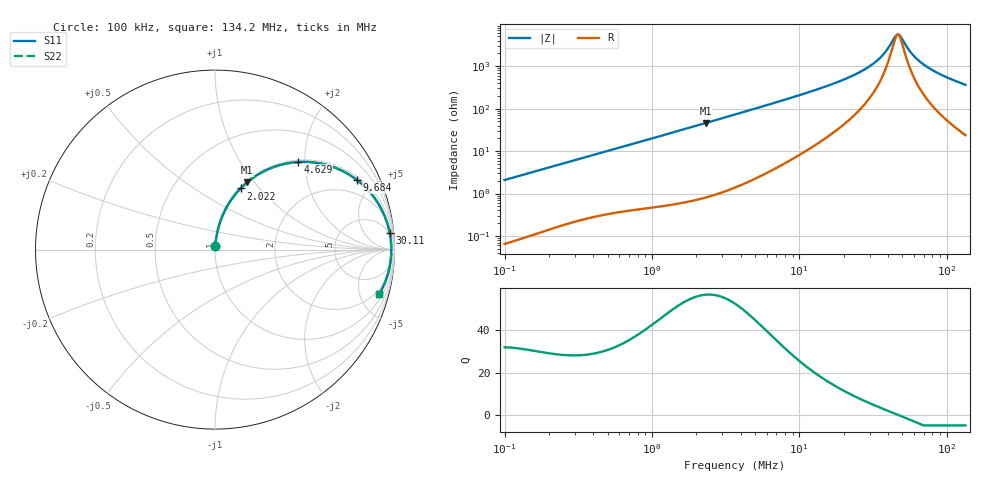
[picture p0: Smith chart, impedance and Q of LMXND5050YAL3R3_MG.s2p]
! LMXND5050YAL3R3_MG  S-PARAMETER MODEL  ( General Type )
! Model Generated by TAIYO YUDEN Corporation (http://www.ty-top.com)
! Version 1.0
! TAIYO YUDEN Control No. 191023NI43SB-FBB
! Copyright(c) 2019 TAIYO YUDEN CO.,LTD. All Rights Reserved.
! Product Description (link to TY-COMPAS)
! https://ds.yuden.co.jp/TYCOMPAS/or/detail?pn=LMXND5050YAL3R3NMG&u=M
! Products Name : Inductors
! Characteristics :
!  Inductance : 3.3 uH , SRF(min) : 32 MHz , DC Resistance(max) : 0.0351 Ohm
!  Rated Current : Saturation :4000 mA , Temp Rise : 3300 mA
!  Case Size : 4.9 x 4.9 / 0.193 x 0.193 [mm/inch] , Thickness : 4.1 / 0.161 [mm/inch]
!  (Conditions: Temperature = 25 degC , DC Bias Current/Voltage = 0A / 0V)
! External Node Assignments :
!  1  o---GGG---o  2
! GND o---------o GND
! Frequency Range : 0.1MHz  -  134.160692MHz  [ 402 STEP ]
# MHz S RI R 50
! Freq[MHz].  S11 Real  S11 Imag  S21 Real  S21 Imag  S12 Real  S12 Imag  S22 Real  S22 Imag
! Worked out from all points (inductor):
!   401 points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, 100 kHz to 134.2 MHz, reference 50 ohm
!   read as one part in series: L = 3.31 uH near 103.7 kHz
!   highest Q = 56.8 at 2.335 MHz (marker M1), where L = 3.15 uH
!   self-resonance near 46.38 MHz
!   S11 on the Smith chart (normalised r, x): 100 kHz: 1.00, +0.04; 2.022 MHz: 1.01, +0.80; 4.629 MHz: 1.04, +1.84; 9.684 MHz: 1.15, +3.98; 30.11 MHz: 5, +20; 134.2 MHz: 1.47, -7.27
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0.1  0.00109 0.0208  0.9989 -0.0208  0.9989 -0.0208  0.00109 0.0208
0.334101  0.00695 0.0672  0.9931 -0.0672  0.9931 -0.0672  0.00695 0.0672
0.638798  0.0196 0.1246  0.9804 -0.1246  0.9804 -0.1246  0.0196 0.1246
1.116232  0.0509 0.2089  0.9491 -0.2089  0.9491 -0.2089  0.0509 0.2089
2.022011  0.1423 0.3405  0.8577 -0.3405  0.8577 -0.3405  0.1423 0.3405
2.335264  0.1801 0.3756  0.8199 -0.3756  0.8199 -0.3756  0.1801 0.3756
3.729338  0.3564 0.4694  0.6436 -0.4694  0.6436 -0.4694  0.3564 0.4694
4.628715  0.46 0.4879  0.54 -0.4879  0.54 -0.4879  0.46 0.4879
6.516624  0.6283 0.47  0.3717 -0.47  0.3717 -0.47  0.6283 0.47
9.683716  0.79 0.3888  0.21 -0.3888  0.21 -0.3888  0.79 0.3888
12.23742  0.8583 0.3254  0.1417 -0.3254  0.1417 -0.3254  0.8583 0.3254
21.00205  0.9482 0.1796  0.0518 -0.1796  0.0518 -0.1796  0.9482 0.1796
30.10531  0.9732 0.0942  0.0268 -0.0942  0.0268 -0.0942  0.9732 0.0942
36.04406  0.9793 0.0548  0.0207 -0.0548  0.0207 -0.0548  0.9793 0.0548
40.88529  0.9816 0.028  0.0184 -0.028  0.0184 -0.028  0.9816 0.028
44.73654  0.9823 0.0091  0.0177 -0.0091  0.0177 -0.0091  0.9823 0.0091
47.21931  0.9824 -0.00223  0.0176 0.00223  0.0176 0.00223  0.9824 -0.00223
48.95057  0.9823 -0.00978  0.0177 0.00978  0.0177 0.00978  0.9823 -0.00978
58.60685  0.9801 -0.0478  0.0199 0.0478  0.0199 0.0478  0.9801 -0.0478
70.16799  0.9747 -0.0869  0.0253 0.0869  0.0253 0.0869  0.9747 -0.0869
93.59314  0.9578 -0.1537  0.0422 0.1537  0.0422 0.1537  0.9578 -0.1537
134.1607  0.916 -0.2466  0.084 0.2466  0.084 0.2466  0.916 -0.2466
